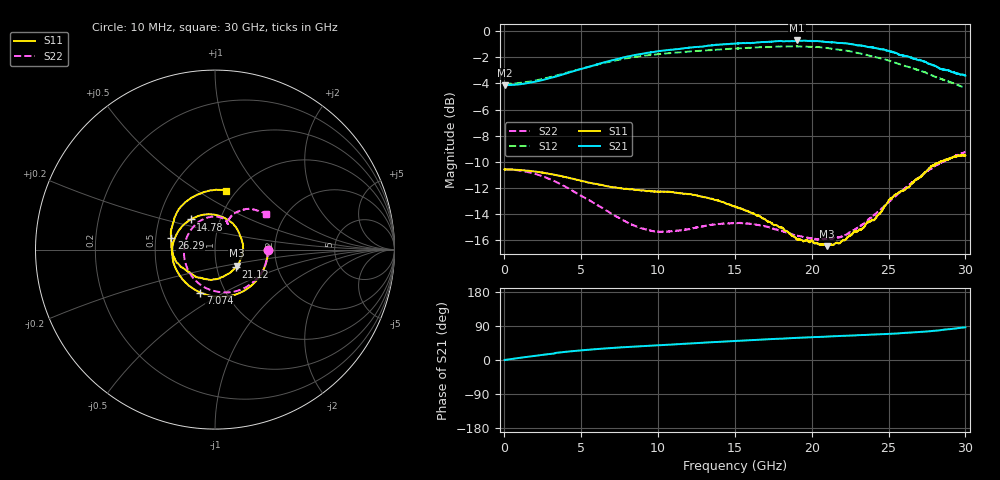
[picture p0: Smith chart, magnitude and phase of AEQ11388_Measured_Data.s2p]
!The following data was pulled from an Agilent PNA
!This sNp file was generated from the data in the RF Test software
!NOTE:  Smoothing/Math/Corrections applied on any given trace ARE included in the data saved here
# MHz S dB R 50
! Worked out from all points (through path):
!   12801 points, 10 MHz to 30 GHz, reference 50 ohm
!   highest |S21| = -0.71 dB at 19.04 GHz (marker M1); lowest = -4.1 dB at 10 MHz (marker M2)
!   lowest |S11| = -16.5 dB at 21 GHz (marker M3), VSWR 1.35, Z = 62.5 - j11.5 ohm
!   |S11| at or under -10 dB: start of sweep to 28.36 GHz
!   |S22| runs from -16.0 to -9.3 dB; largest |S21 - S12| = 1.7
!   S11 on the Smith chart (normalised r, x): 10 MHz: 1.84, -0.00; 7.074 GHz: 0.76, -0.39; 14.78 GHz: 0.73, +0.26; 21.12 GHz: 1.23, -0.25; 26.29 GHz: 0.60, +0.08; 30 GHz: 0.90, +0.67
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10  -10.58 -0.2  -4.15 0.0  -4.02 -0.1  -10.59 -0.1
1350.178  -10.67 -22.0  -4.00 7.7  -3.91 -10.2  -10.75 -22.9
2784.075  -10.91 -45.1  -3.65 15.1  -3.57 -21.8  -11.26 -47.8
5009.896  -11.47 -79.2  -2.89 25.4  -2.88 -42.5  -12.62 -88.0
7074.051  -11.95 -108.8  -2.22 31.9  -2.29 -64.1  -14.04 -129.0
8589.951  -12.17 -130.4  -1.81 35.6  -1.96 -80.8  -14.97 -160.6
10007.45  -12.29 -150.9  -1.53 38.9  -1.75 -96.7  -15.36 170.8
12310.59  -12.55 172.3  -1.22 44.1  -1.53 -122.6  -15.09 130.2
14782.42  -13.34 128.7  -0.96 49.6  -1.35 -150.7  -14.71 96.5
15005  -13.44 124.1  -0.94 50.2  -1.33 -153.2  -14.69 94.2
17003.55  -14.45 82.4  -0.83 54.4  -1.22 -176.5  -14.95 75.7
18050.86  -15.04 57.0  -0.75 56.3  -1.17 171.1  -15.31 69.2
19039.59  -15.99 29.8  -0.71 58.5  -1.14 159.1  -15.66 66.1
20004.89  -16.03 -0.9  -0.76 60.1  -1.20 147.1  -15.87 63.8
21003  -16.47 -36.9  -0.83 61.9  -1.29 134.5  -15.89 63.6
21115.46  -16.39 -40.6  -0.83 62.0  -1.31 133.1  -15.91 63.3
23029.67  -15.27 -107.7  -1.09 65.5  -1.68 109.1  -15.04 65.1
25002.45  -12.94 -161.5  -1.51 68.9  -2.25 84.8  -13.10 62.8
26293.42  -11.95 165.0  -1.94 72.0  -2.73 69.5  -11.83 57.4
27755.44  -10.38 131.7  -2.55 76.3  -3.35 52.3  -10.53 49.8
28823.83  -9.84 105.1  -2.98 80.9  -3.82 41.0  -9.83 42.4
30000  -9.53 79.0  -3.40 86.2  -4.34 28.7  -9.26 35.0
